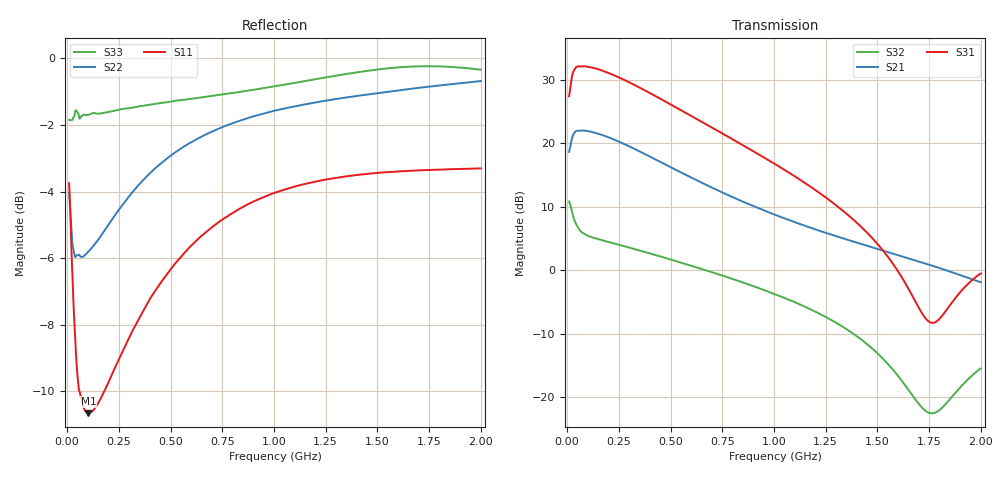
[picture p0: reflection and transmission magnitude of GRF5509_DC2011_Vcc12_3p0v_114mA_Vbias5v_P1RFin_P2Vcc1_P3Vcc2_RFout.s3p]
!Keysight Technologies,N5244B,MY57181157,A.18.40.03
!Date: Wednesday, April 29, 2026 14:32:45
!Correction: S11(C  3-Port  )
!S12(C  3-Port  )
!S13(C  3-Port  )
!S21(C  3-Port  )
!S22(C  3-Port  )
!S23(C  3-Port  )
!S31(C  3-Port  )
!S32(C  3-Port  )
!S33(C  3-Port  )
!S3P File: Measurements: <S11,S12,S13>,
!<S21,S22,S23>,
!<S31,S32,S33>:
# Hz S  dB  R 50
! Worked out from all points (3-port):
!   1991 points, 10 MHz to 2 GHz, reference 50 ohm
!   strongest paths, dB at 10 MHz, 507 MHz, 1.005 GHz, 1.503 GHz, 2 GHz:
!     S31: 27.4, 26.0, 16.7, 4.0, -0.5
!     S21: 18.7, 16.1, 8.7, 3.3, -1.9
!     S32: 10.8, 1.6, -3.8, -13.2, -15.5
!   lowest |S11| = -10.7 dB at 103 MHz (marker M1), VSWR 1.83, Z = 31.3 - j15.4 ohm
!   |S11| at or under -10 dB: 58.66 MHz to 180.1 MHz (121.4 MHz wide, 102 % of centre)
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1e7  -3.75 -52.8  -22.09 -33.7  -55.06 -96.7
     18.68 -136.5  -4.04 -77.5  -32.05 -85.7
     27.43 77.1  10.82 -174.9  -1.84 -116.8
3e7  -7.19 -89.1  -26.57 -42.7  -64.28 118.1
     21.39 -161.6  -5.73 -121.6  -43.44 145.1
     31.27 31.8  8.44 161.3  -1.79 -150.0
4.4e7  -8.98 -106.0  -28.64 -42.2  -65.70 -45.2
       21.96 -172.8  -5.93 -135.9  -43.00 -39.4
       32.02 15.7  7.28 157.7  -1.56 -159.8
1.03e8  -10.67 -129.7  -32.27 -30.8  -73.15 -27.1
        21.92 163.7  -5.81 -155.6  -50.98 31.7
        32.08 -16.4  5.39 153.6  -1.69 -170.2
1.7e8  -10.13 -135.8  -33.22 -24.4  -71.81 69.7
       21.33 146.3  -5.27 -160.2  -45.48 45.2
       31.49 -38.4  4.71 146.8  -1.64 -172.7
2.5e8  -9.05 -138.5  -33.70 -22.6  -67.01 61.2
       20.29 129.5  -4.55 -163.0  -42.53 43.2
       30.42 -59.4  4.02 137.6  -1.54 -173.5
4.74e8  -6.56 -144.5  -34.69 -24.4  -60.65 83.9
        16.69 95.4  -3.05 -170.1  -39.72 33.3
        26.63 -104.7  1.94 113.5  -1.32 -173.6
6.72e8  -5.22 -150.3  -35.53 -26.8  -57.99 83.3
        13.47 75.7  -2.28 -175.7  -39.25 28.7
        23.01 -134.6  -0.03 95.0  -1.15 -173.4
1.005e9  -4.04 -159.1  -36.78 -28.2  -54.56 86.0
         8.74 54.5  -1.57 177.4  -39.74 30.3
         16.74 -174.2  -3.77 67.5  -0.84 -173.6
2e9  -3.31 -177.9  -39.63 -43.8  -47.99 92.2
     -1.90 11.0  -0.68 156.3  -34.79 70.8
     -0.53 -126.3  -15.52 122.0  -0.34 172.2
